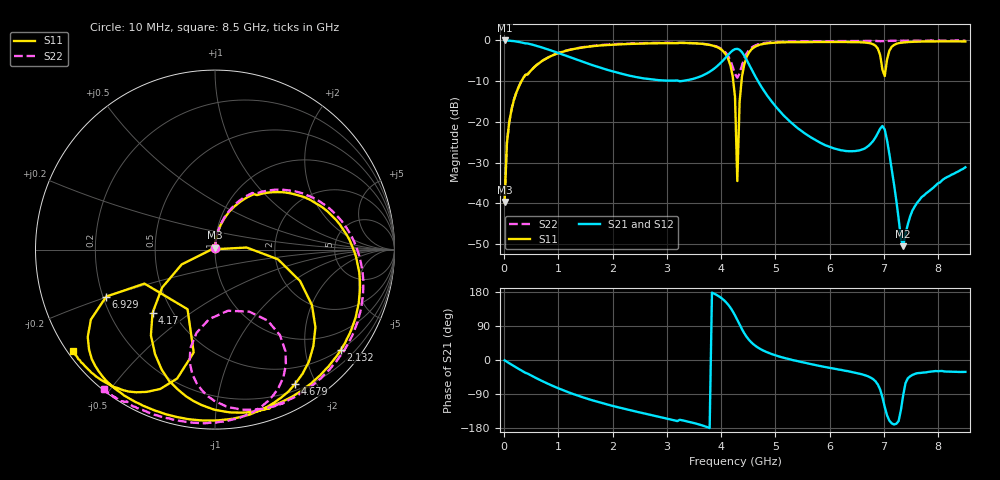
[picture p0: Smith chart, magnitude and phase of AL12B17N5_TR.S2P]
!AVX CORPORATION
!PART NUMBER AL12B17N5_TR
!DESCRIPTION: AIR CORE INDUCTOR, 17.5nH, 6 TURNS
!Agilent Technologies,E5071C,MY46102230,A.09.54
!Date: Mon Sep 03 15:55:19 2012
!Data & Calibration Information:
!Freq	S11:SOLT2(ON)	S21:SOLT2(ON)	S12:SOLT2(ON)	S22:SOLT2(ON)
# Hz S RI R 50
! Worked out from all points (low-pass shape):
!   201 points, 10 MHz to 8.5 GHz, reference 50 ohm
!   highest |S21| = -0.01 dB at 10 MHz (marker M1); lowest = -50.5 dB at 7.354 GHz (marker M2)
!   |S21| within 3 dB of the highest: start of sweep to 982.8 MHz; 4.167 GHz to 4.389 GHz (221.9 MHz wide, 5.19 % of centre)
!   lowest |S11| = -39.7 dB at 10 MHz (marker M3), VSWR 1.02, Z = 50 + j1.04 ohm
!   |S11| at or under -10 dB: start of sweep to 321.2 MHz; 4.223 GHz to 4.375 GHz (152.6 MHz wide, 3.55 % of centre)
!   |S22| runs from -39.2 to 0.0 dB; largest |S21 - S12| = 0.0083
!   S11 on the Smith chart (normalised r, x): 10 MHz: 1.00, +0.02; 2.132 GHz: 0.49, -2.77; 4.17 GHz: 0.39, -0.36; 4.679 GHz: 0.28, -1.73; 6.929 GHz: 0.21, -0.20; 8.5 GHz: 0.02, -0.32
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1e7  0.000242 0.0104  0.9992 -0.0161  0.9937 -0.0224  0.000362 0.011
5.245e7  0.0048 0.0547  0.994 -0.0821  0.9993 -0.0817  0.00476 0.0551
9.49e7  0.0158 0.0976  0.9826 -0.1465  0.9841 -0.148  0.0156 0.098
3.0715e8  0.1433 0.2684  0.8467 -0.426  0.8484 -0.4281  0.1363 0.273
1.4533e9  0.8058 -0.1583  -0.0811 -0.5397  -0.0816 -0.5401  0.819 -0.106
2.1325e9  0.6992 -0.5606  -0.2318 -0.319  -0.2321 -0.3192  0.7441 -0.5192
2.85415e9  0.4207 -0.8243  -0.2812 -0.1632  -0.2815 -0.1629  0.4894 -0.794
3.8305e9  -0.0767 -0.8652  -0.4313 0.0169  -0.4315 0.017  0.0593 -0.8724
4.1701e9  -0.3482 -0.3531  -0.5305 0.474  -0.5299 0.4737  -0.1372 -0.5487
4.255e9  -0.1858 -0.0828  -0.3658 0.6915  -0.3651 0.6919  -0.0327 -0.3876
4.29745e9  -0.0188 0.000844  -0.2167 0.7593  -0.2166 0.7594  0.0715 -0.3407
4.3399e9  0.1764 0.0116  -0.0474 0.7654  -0.047 0.766  0.1907 -0.3455
4.38235e9  0.3508 -0.0539  0.104 0.7101  0.1045 0.7106  0.2927 -0.3951
4.6795e9  0.4474 -0.7466  0.2661 0.1701  0.2664 0.1701  0.2965 -0.843
5.6983e9  -0.2345 -0.9272  0.0606 -0.0132  0.0605 -0.0131  -0.2128 -0.9504
6.6322e9  -0.6291 -0.7038  0.0361 -0.0296  0.036 -0.0296  -0.4432 -0.8772
6.92935e9  -0.6055 -0.2613  0.0174 -0.0809  0.0171 -0.0808  -0.4871 -0.8494
7.01425e9  -0.1528 -0.3322  -0.0451 -0.0666  -0.0451 -0.0666  -0.4915 -0.8454
7.09915e9  -0.2107 -0.7182  -0.0379 -0.0138  -0.0376 -0.0138  -0.5054 -0.8493
7.35385e9  -0.5434 -0.771  -0.00015 -0.00298  -2.7e-05 -0.00318  -0.5378 -0.8368
7.60855e9  -0.6474 -0.7168  0.00832 -0.0058  0.00817 -0.00567  -0.5627 -0.8213
8.5e9  -0.7899 -0.5629  0.0237 -0.0144  0.0235 -0.0142  -0.6208 -0.7755
